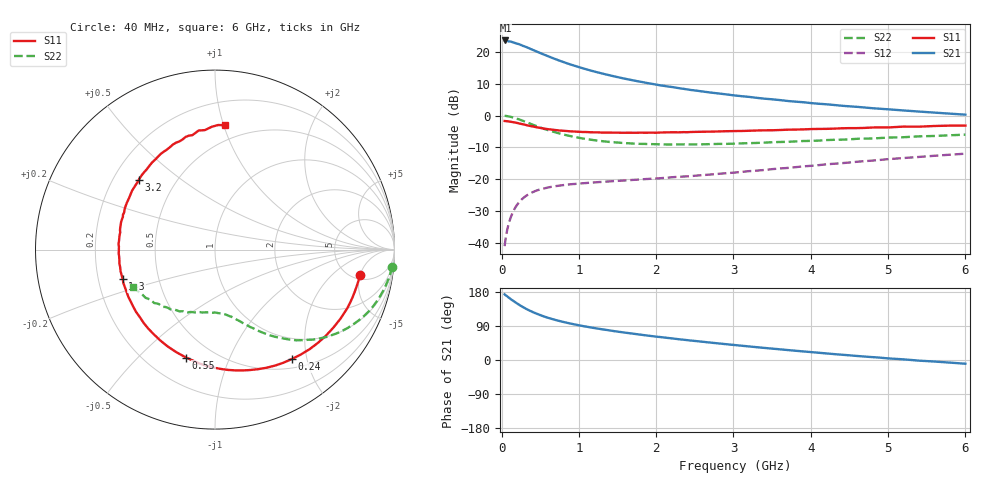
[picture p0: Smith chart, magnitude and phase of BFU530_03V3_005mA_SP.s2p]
! Filename:  P:\Prog\Test\Noise\ATS_data\Testdata_Net\03 Spar\BFU530_APG2013_40_A05_03p3V_005mA_SP_CM01_D.s2p
! Date/Time: Fri 26/Apr/2013 13:03:16
! BFU530_APG2013_40_A05_03p3V_1to25mA_SP_CM01_Bias4_R.s2p
! MDIF S-parameter v. bias file
! BFU530_APG2013_40_A05_03p3V_1to25mA_SP_CM01
! Date/time Wed Apr 24 18:17:07 2013
! VAR V_out= 3.3000
! VAR I_out= 4.9950
! VAR V_in= 0.8220
! VAR I_in= 0.0552
! Device data file deembeded for feedlines and parallel
! Original file: \03 Spar\BFU530_APG2013_40_A05_03p3V_005mA_SP_CM01_R.s2p
! Feed-files: PR047V01_250413_Feed1.s2p, PR047V01_250413_Feed2.s2p
! Parallel-file: PR047V01_250413_Par.s2p
# MHz S MA R 50
!  Freq-MHz  S11-mag  S11-arg  S21-mag  S21-arg  S12-mag  S12-arg  S22-mag  S22-arg
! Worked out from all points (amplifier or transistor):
!   98 points, 40 MHz to 6 GHz, reference 50 ohm
!   highest |S21| = 23.6 dB at 50 MHz (marker M1)
!   |S21| within 3 dB of that: start of sweep to 408.8 MHz
!   unconditionally stable (mu >= 1): 2.226 GHz to 4.51 GHz
!   at 300 MHz: K = 0.19, MSG = 23.7 dB, |S12| = -25.6 dB
!   at 1.6 GHz: K = 0.84, MSG = 16.0 dB, |S12| = -20.4 dB
!   at 6 GHz: K = 0.87, MSG = 6.1 dB, |S12| = -12.0 dB
!   S11 on the Smith chart (normalised r, x): 40 MHz: 5.85, -4.99; 240 MHz: 0.64, -1.74; 550 MHz: 0.36, -0.70; 1.3 GHz: 0.31, -0.14; 3.2 GHz: 0.31, +0.36; 6 GHz: 0.38, +1.01
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40  0.821 -9.7  15.16 173.4  0.008817 84.6  0.9896 -5.5
50  0.8181 -12.2  15.17 171.1  0.0109 83.3  0.988 -6.8
140  0.7899 -33.4  14.3 157.6  0.02895 72.4  0.9393 -19.1
180  0.774 -42.2  13.76 152.1  0.03601 67.9  0.9094 -24.0
240  0.745 -55.0  13.04 144.1  0.04509 62.0  0.8587 -30.6
320  0.7078 -70.3  11.96 134.8  0.05478 55.4  0.7885 -38.1
360  0.6905 -77.2  11.38 130.8  0.05874 52.6  0.7553 -41.4
440  0.6593 -89.8  10.35 123.4  0.06517 48.0  0.6921 -46.8
550  0.6226 -105.0  9.098 114.7  0.07127 43.1  0.6167 -53.1
650  0.6005 -116.1  8.123 108.4  0.07592 40.0  0.5658 -57.5
750  0.5822 -125.9  7.3 102.9  0.07913 37.8  0.5226 -61.1
900  0.5628 -138.3  6.316 95.8  0.08308 35.5  0.4729 -65.6
1050  0.5513 -148.6  5.545 89.7  0.08597 34.2  0.4358 -69.4
1300  0.54 -162.4  4.588 81.1  0.09045 33.3  0.3958 -74.6
1600  0.5355 -176.2  3.786 72.1  0.09535 33.4  0.3687 -80.2
2050  0.5404 168.4  2.993 60.6  0.1033 34.8  0.3523 -88.2
2450  0.5512 155.9  2.524 51.3  0.1114 36.3  0.3511 -95.6
3100  0.5717 139.3  2.019 37.8  0.1296 38.6  0.365 -106.6
3200  0.576 137.5  1.966 35.8  0.1334 38.9  0.3679 -108.0
4100  0.616 117.7  1.533 19.2  0.1658 38.5  0.4031 -123.9
5200  0.6696 97.8  1.202 1.7  0.2146 34.0  0.456 -142.4
6000  0.6951 85.4  1.033 -9.8  0.2513 28.2  0.5004 -155.5
